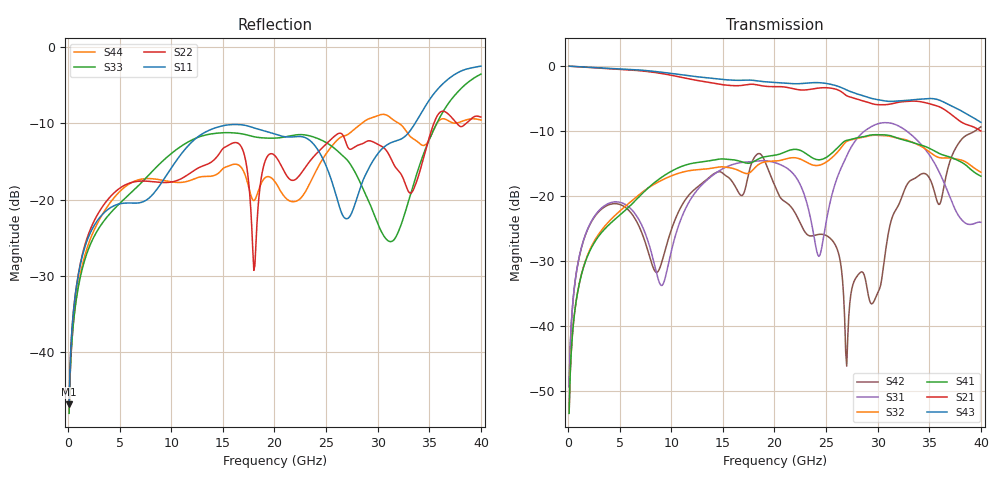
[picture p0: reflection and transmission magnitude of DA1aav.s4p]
! ADC12DJ2700AAV, ADC12DJ3200AAV, ADC08DJ3200AAV
! 144 pin AAV package
! Texas Instruments 4/21/2021
! Single-ended  S-parameters
! PORT#  PORT_NAME  NET_NAME
! PORT1:  DAxN.DIEBUMP DAxN
! PORT2:  DAxN.BGA  DAxN
! PORT3:  DAxP.DIEBUMP DAxP
! PORT4:  DAxP.BGA  DAxP
! Touchstone Ver. 1.0
! Number of ports is 4
# Hz	S	MA	R	50.000000
! SCATTERING PARAMETERS  :
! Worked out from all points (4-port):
!   400 points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, 100 MHz to 40 GHz, reference 50 ohm
!   strongest paths, dB at 100 MHz, 10.1 GHz, 20.1 GHz, 30.1 GHz, 40 GHz:
!     S43: 0.0, -1.2, -2.5, -5.2, -8.7
!     S21: 0.0, -1.4, -3.2, -6.0, -10.0
!     S41: -53.4, -16.1, -13.7, -10.6, -16.9
!     S32: -53.4, -16.8, -14.6, -10.7, -16.3
!     S31: -49.4, -27.9, -14.9, -8.8, -24.1
!     S42: -49.4, -24.8, -18.7, -34.5, -9.4
!   lowest |S11| = -46.8 dB at 100 MHz (marker M1), VSWR 1.01, Z = 50.2 + j0.416 ohm
!   |S11| at or under -10 dB: start of sweep to 33.63 GHz
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1e8  0.004594 64.4  0.9978 -1.5  0.003408 84.9  0.002128 -97.2
     0.9978 -1.5  0.004597 63.7  0.002128 -97.1  0.003405 84.7
     0.003408 84.9  0.002128 -97.1  0.003999 62.7  0.9979 -1.4
     0.002128 -97.2  0.003405 84.7  0.9979 -1.4  0.004014 61.6
2.7e9  0.07071 46.5  0.9674 -38.4  0.0725 46.1  0.04582 -143.9
       0.9674 -38.4  0.07653 26.1  0.04725 -142.6  0.07148 41.9
       0.0725 46.1  0.04725 -142.6  0.0604 57.9  0.9715 -35.9
       0.04582 -143.9  0.07148 41.9  0.9715 -35.9  0.06704 19.7
9.9e9  0.1575 29.9  0.8524 -137.8  0.03472 77.9  0.1534 113.2
       0.8524 -137.8  0.1301 -69.9  0.1418 108.7  0.05193 58.8
       0.03472 77.9  0.1418 108.7  0.1978 26.9  0.88 -128.5
       0.1534 113.2  0.05193 58.8  0.88 -128.5  0.1311 -89.2
1.86e10  0.287 -58.3  0.7092 114.1  0.1868 17.5  0.1956 -21.7
         0.7092 114.1  0.1215 -113.3  0.1776 -12.1  0.2114 -34.5
         0.1868 17.5  0.1776 -12.1  0.2545 -43.8  0.764 126.5
         0.1956 -21.7  0.2114 -34.5  0.764 126.5  0.1225 -135.9
2.43e10  0.2067 -125.0  0.6774 41.6  0.03434 -144.3  0.1899 -106.2
         0.6774 41.6  0.2076 41.9  0.1722 -89.4  0.05067 66.5
         0.03434 -144.3  0.1722 -89.4  0.2495 -89.0  0.745 55.0
         0.1899 -106.2  0.05067 66.5  0.745 55.0  0.1671 16.3
2.7e10  0.07503 131.0  0.5913 -1.4  0.2037 92.4  0.2681 -139.4
        0.5913 -1.4  0.2288 -42.9  0.263 -119.5  0.004906 -178.5
        0.2037 92.4  0.263 -119.5  0.1833 -124.1  0.653 15.6
        0.2681 -139.4  0.004906 -178.5  0.653 15.6  0.2646 -47.2
4e10  0.7472 -85.0  0.3161 -173.4  0.06271 9.4  0.1421 -11.4
      0.3161 -173.4  0.3473 -90.7  0.1525 17.7  0.3406 77.0
      0.06271 9.4  0.1525 17.7  0.6626 -35.1  0.3691 -150.2
      0.1421 -11.4  0.3406 77.0  0.3691 -150.2  0.3322 -122.3
